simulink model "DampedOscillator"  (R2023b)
settings: Solver=ode45  StartTime=0.0  StopTime=10  RelTol=1e-3

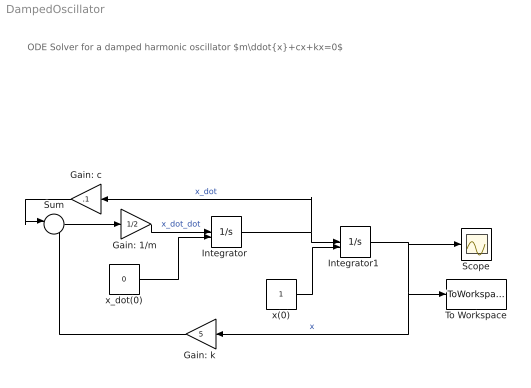
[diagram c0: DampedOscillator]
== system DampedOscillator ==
  note: ODE Solver for a damped harmonic oscillator $m\ddot{x}+cx+kx=0$
  "Gain: 1/m " : Gain  Gain=1/2
  Gain: c : Gain  Gain=.1
  "Gain: k " : Gain  Gain=5
  "Integrator " : Integrator  InitialConditionSource=external
  "Integrator1 " : Integrator  InitialConditionSource=external
  Scope : Scope
  Sum : Sum  Inputs=|--
  To Workspace : ToWorkspace  VariableName=sol  SaveFormat=Timeseries  SampleTime=-1
  x(0) : Constant
  x_dot(0) : Constant  Value=0
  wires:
  x(0)/1 -> "Integrator1 "/2
  "Integrator "/1 -> Gain: c/1, "Integrator1 "/1  "x_dot"
  Sum/1 -> "Gain: 1/m "/1
  Gain: c/1 -> Sum/1
  "Gain: 1/m "/1 -> "Integrator "/1  "x_dot_dot"
  "Gain: k "/1 -> Sum/2
  "Integrator1 "/1 -> Scope/1, "Gain: k "/1, To Workspace/1  "x"
  x_dot(0)/1 -> "Integrator "/2
